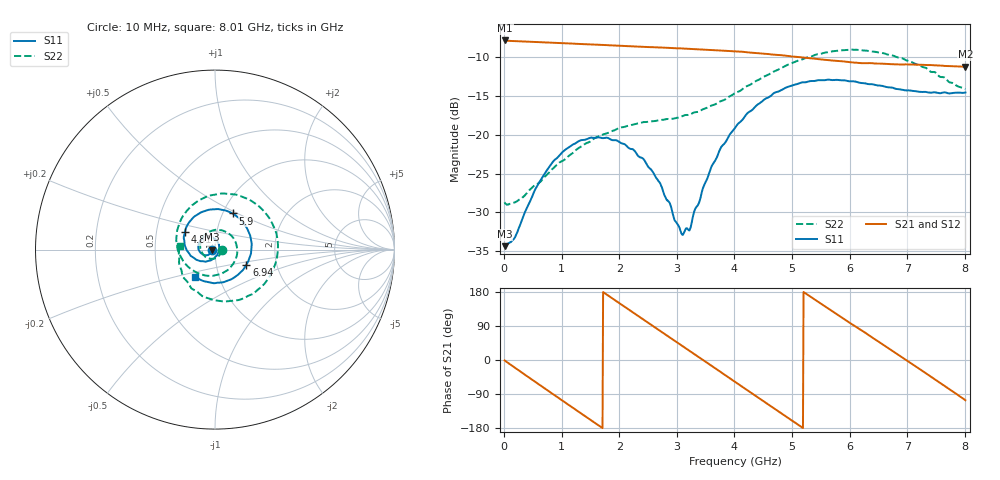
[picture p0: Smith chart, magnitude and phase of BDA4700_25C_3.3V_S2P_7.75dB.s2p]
!Agilent Technologies,E5071B,MY42404982,A.09.10
!Date: Mon Oct 20 18:06:15 2025
!Data & Calibration Information:
!Freq	S11:SOLT2(ON)	S21:SOLT2(ON)	S12:SOLT2(ON)	S22:SOLT2(ON)
# Hz S RI R 50
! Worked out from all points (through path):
!   801 points, 10 MHz to 8.01 GHz, reference 50 ohm
!   highest |S21| = -7.86 dB at 20 MHz (marker M1); lowest = -11.2 dB at 8.01 GHz (marker M2)
!   group delay of S21, straight-line fit = 286 ps
!   lowest |S11| = -34.3 dB at 10 MHz (marker M3), VSWR 1.04, Z = 48.1 - j0.086 ohm
!   |S11| at or under -10 dB: start of sweep to end of sweep
!   |S22| runs from -29.0 to -9.0 dB; largest |S21 - S12| = 0.0047
!   S11 on the Smith chart (normalised r, x): 10 MHz: 0.96, -0.00; 4.81 GHz: 0.70, +0.14; 5.9 GHz: 1.11, +0.47; 6.94 GHz: 1.40, -0.24; 8.01 GHz: 0.77, -0.24
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1e7  -0.0192 -0.000893  0.4041 -0.00876  0.4043 -0.00907  0.0367 -0.00272
2e7  -0.0195 -0.00158  0.4041 -0.0158  0.4038 -0.0169  0.0361 -0.00308
1.9e8  -0.0196 -0.00973  0.3751 -0.1402  0.375 -0.1405  0.0321 -0.0178
7.2e8  -0.048 -0.0314  0.0922 -0.3817  0.0924 -0.3818  -0.0169 -0.0516
1.02e9  -0.0742 -0.0233  -0.1186 -0.3701  -0.1185 -0.3699  -0.0579 -0.0358
1.35e9  -0.0924 0.00416  -0.3034 -0.2347  -0.3035 -0.235  -0.0825 0.0175
1.93e9  -0.0682 0.0622  -0.3463 0.1441  -0.3462 0.1441  -0.00989 0.1069
2.32e9  -0.0255 0.0691  -0.1683 0.3289  -0.168 0.3288  0.0792 0.0877
2.68e9  0.0112 0.0492  0.0639 0.3591  0.0633 0.359  0.1236 0.00585
3.12e9  0.0227 -0.00516  0.2958 0.2028  0.2948 0.2035  0.0813 -0.1054
3.23e9  0.0174 -0.0176  0.3283 0.1408  0.3282 0.1402  0.0553 -0.123
3.55e9  -0.0135 -0.0533  0.3472 -0.0602  0.3472 -0.061  -0.0386 -0.146
4.01e9  -0.0929 -0.0603  0.1845 -0.2908  0.1851 -0.2903  -0.1687 -0.0757
4.4e9  -0.1561 -0.00573  -0.0468 -0.3322  -0.0465 -0.3329  -0.2155 0.0611
4.81e9  -0.1676 0.0963  -0.2511 -0.2065  -0.2497 -0.2082  -0.1534 0.2206
5.35e9  -0.0699 0.2105  -0.2979 0.085  -0.2983 0.0832  0.0827 0.3094
5.9e9  0.0986 0.2012  -0.0933 0.2811  -0.0942 0.2802  0.3146 0.1538
6.28e9  0.18 0.1155  0.0933 0.2732  0.0971 0.2708  0.3448 -0.0473
6.68e9  0.2016 -0.00889  0.2457 0.1445  0.2464 0.144  0.2381 -0.2241
6.94e9  0.1751 -0.0836  0.2824 0.022  0.2824 0.0201  0.1215 -0.2823
7.53e9  0.0302 -0.1836  0.1551 -0.2324  0.1543 -0.2326  -0.143 -0.1962
8.01e9  -0.1092 -0.152  -0.0763 -0.2632  -0.0756 -0.2635  -0.1964 0.0199
